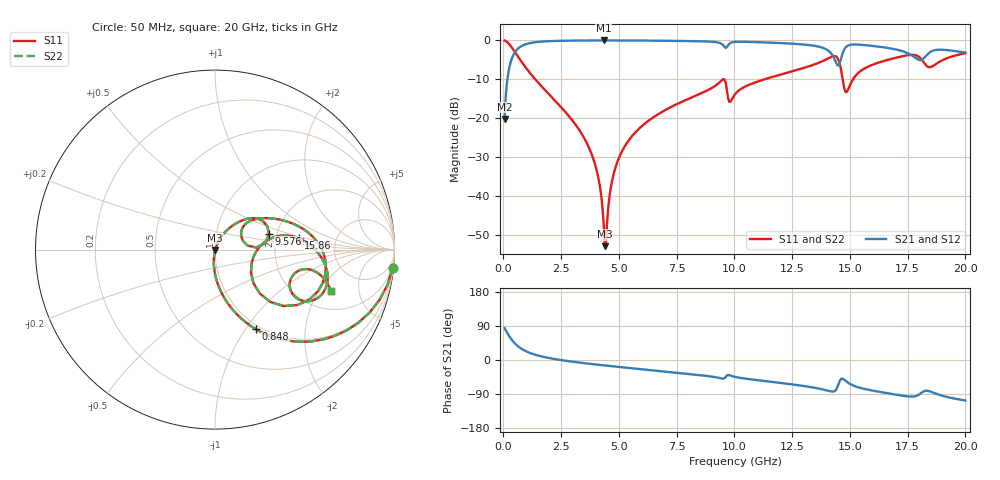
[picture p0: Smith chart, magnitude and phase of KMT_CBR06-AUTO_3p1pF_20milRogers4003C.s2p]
! Data measured by Modelithics Inc. support@modelithics.com 813-866-6335
! KEMET CBR06-AUTO 3.1pF, Pad Width= 0.851mm, Pad Length= 0.64mm, Pad Gap= 0.62mm, 20mil Rogers 4003C substrate Data, January 2022
# hz S ma R 50
! 2 Port Network Data from SP1.SP block
! freq  magS11  angS11  magS21  angS21  magS12  angS12  magS22  angS22
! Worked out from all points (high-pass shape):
!   401 points, 50 MHz to 20 GHz, reference 50 ohm
!   highest |S21| = -0.02 dB at 4.339 GHz (marker M1); lowest = -20.2 dB at 50 MHz (marker M2)
!   |S21| within 3 dB of the highest: 501.8 MHz to 14.14 GHz (13.64 GHz wide, 186 % of centre); 14.7 GHz to 17.39 GHz (2.69 GHz wide, 16.8 % of centre)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
!   lowest |S11| = -52.8 dB at 4.389 GHz (marker M3), VSWR 1.00, Z = 50.2 - j0.171 ohm
!   |S11| at or under -10 dB: 1.381 GHz to 9.505 GHz (8.124 GHz wide, 149 % of centre); 9.551 GHz to 11.29 GHz (1.743 GHz wide, 16.7 % of centre); 14.69 GHz to 15.13 GHz (446.5 MHz wide, 2.99 % of centre)
!   |S22| runs from -52.8 to 0.0 dB; largest |S21 - S12| = 0
!   S11 on the Smith chart (normalised r, x): 50 MHz: 1, -20; 848 MHz: 0.95, -1.12; 9.576 GHz: 1.82, +0.35; 15.86 GHz: 2.70, +0.44; 20 GHz: 2.99, -2.57
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5e7  0.9952 -5.8  0.09798 84.2  0.09798 84.2  0.9952 -5.8
3.4925e8  0.822 -35.8  0.5686 54.1  0.5686 54.1  0.822 -35.8
8.48e8  0.5 -62.7  0.8649 27.2  0.8649 27.2  0.5 -62.7
3.391625e9  0.06322 -96.1  0.9962 -7.6  0.9962 -7.6  0.06322 -96.1
4.04e9  0.02137 -97.2  0.9978 -12.2  0.9978 -12.2  0.02137 -97.2
4.33925e9  0.004471 -78.8  0.9979 -14.2  0.9979 -14.2  0.004471 -78.8
4.389125e9  0.002303 -47.6  0.9979 -14.5  0.9979 -14.5  0.002303 -47.6
4.73825e9  0.01769 66.8  0.9977 -16.7  0.9977 -16.7  0.01769 66.8
5.087375e9  0.0356 67.8  0.9971 -18.9  0.9971 -18.9  0.0356 67.8
6.73325e9  0.1148 59.9  0.9906 -28.8  0.9906 -28.8  0.1148 59.9
9.576125e9  0.3136 16.2  0.8217 -47.8  0.8217 -47.8  0.3136 16.2
9.8255e9  0.164 27.0  0.9265 -41.0  0.9265 -41.0  0.164 27.0
1.0025e10  0.2037 39.2  0.9566 -44.5  0.9566 -44.5  0.2037 39.2
1.336662e10  0.4807 15.9  0.8599 -72.2  0.8599 -72.2  0.4807 15.9
1.426438e10  0.625 -8.7  0.6322 -83.3  0.6322 -83.3  0.625 -8.7
1.456362e10  0.4953 -39.4  0.5131 -54.7  0.5131 -54.7  0.4953 -39.4
1.486288e10  0.2182 -10.3  0.8378 -57.3  0.8378 -57.3  0.2182 -10.3
1.586038e10  0.4713 7.7  0.8566 -79.3  0.8566 -79.3  0.4713 7.7
1.670825e10  0.5697 -1.3  0.7938 -88.5  0.7938 -88.5  0.5697 -1.3
1.8005e10  0.6094 -27.8  0.5608 -90.6  0.5608 -90.6  0.6094 -27.8
1.8404e10  0.4549 -23.5  0.6821 -81.8  0.6821 -81.8  0.4549 -23.5
2e10  0.6845 -19.5  0.6992 -107.0  0.6992 -107.0  0.6845 -19.5
